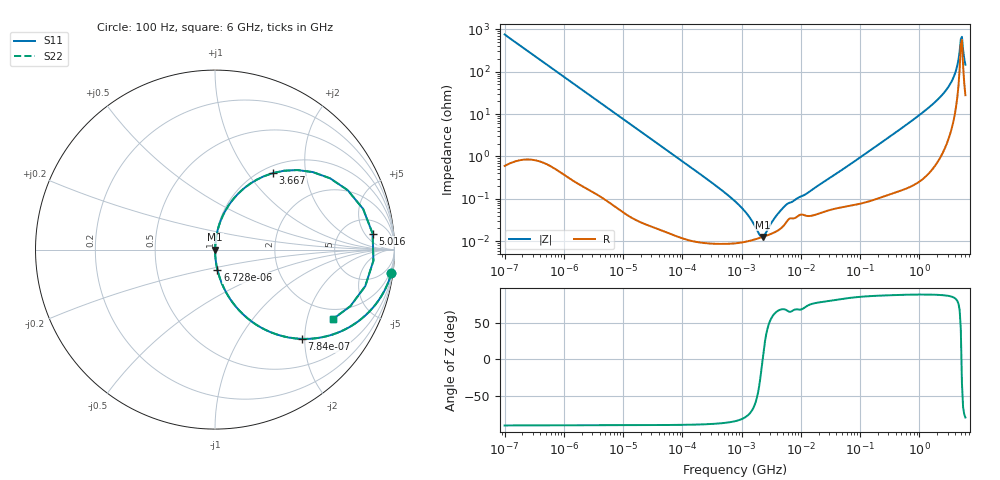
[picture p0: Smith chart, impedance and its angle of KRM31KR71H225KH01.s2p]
!Murata Part Number: KRM31KR71H225KH01
!These Parameters are Measured in Series Mode Connection
!Data Generated on Jan 08, 2026
!  o--ll--o
!Port1  Port2
!  o------o
!Operation Temp=25[degC], DC Bias Voltage=0[V]
!Freq. Start=100[Hz] Stop=6[GHz] 401[Steps]
# Hz S RI R 50
!Freq.(Hz) S11(Real) S11(Imag) S21(Real) S21(Imag) S12(Real) S12(Imag) S22(Real) S22(Imag)
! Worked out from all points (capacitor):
!   401 points, 100 Hz to 6 GHz, reference 50 ohm
!   read as one part in series: C = 2.11 uF near 109 Hz
!   lowest |Z| = 12.6 mohm at 2.269 MHz (marker M1)
!   series resonance near 2.264 MHz, so ESL is about 2.3 nH
!   S11 on the Smith chart (normalised r, x): 100 Hz: 1, -15; 784 Hz: 1.01, -1.93; 6.728 kHz: 1.00, -0.23; 3.667 GHz: 1.11, +1.33; 5.016 GHz: 10, +8; 6 GHz: 1.56, -2.88
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100  0.9827 -0.13  0.0173 0.13  0.0173 0.13  0.9827 -0.13
293  0.8688 -0.336  0.1312 0.336  0.1312 0.336  0.8688 -0.336
784  0.4836 -0.4973  0.5164 0.4973  0.5164 0.4973  0.4836 -0.4973
2008  0.1269 -0.3302  0.8731 0.3302  0.8731 0.3302  0.1269 -0.3302
6728  0.0134 -0.1121  0.9866 0.1121  0.9866 0.1121  0.0134 -0.1121
40335  0.000553 -0.019  0.9994 0.019  0.9994 0.019  0.000553 -0.019
774597  9e-05 -0.000875  0.9999 0.000875  0.9999 0.000875  9e-05 -0.000875
1212075  9.85e-05 -0.000446  0.9999 0.000446  0.9999 0.000446  9.85e-05 -0.000446
1983483  0.000119 -8.69e-05  0.9999 8.69e-05  0.9999 8.69e-05  0.000119 -8.69e-05
2268635  0.000126 1.5e-06  0.9999 -1.5e-06  0.9999 -1.5e-06  0.000126 1.5e-06
5311619  0.000247 0.000619  0.9998 -0.000619  0.9998 -0.000619  0.000247 0.000619
1.555665e7  0.000404 0.00159  0.9996 -0.00159  0.9996 -0.00159  0.000404 0.00159
3.124326e8  0.00209 0.0288  0.9979 -0.0288  0.9979 -0.0288  0.00209 0.0288
9.569533e8  0.0104 0.089  0.9896 -0.089  0.9896 -0.089  0.0104 0.089
2.048624e9  0.0528 0.2072  0.9472 -0.2072  0.9472 -0.2072  0.0528 0.2072
2.931063e9  0.1454 0.3272  0.8546 -0.3272  0.8546 -0.3272  0.1454 0.3272
3.666503e9  0.3223 0.4263  0.6777 -0.4263  0.6777 -0.4263  0.3223 0.4263
4.385646e9  0.6412 0.3973  0.3588 -0.3973  0.3588 -0.3973  0.6412 0.3973
4.796499e9  0.8253 0.2263  0.1747 -0.2263  0.1747 -0.2263  0.8253 0.2263
5.016141e9  0.8781 0.0895  0.1219 -0.0895  0.1219 -0.0895  0.8781 0.0895
5.486059e9  0.837 -0.2038  0.163 0.2038  0.163 0.2038  0.837 -0.2038
6e9  0.6554 -0.3883  0.3446 0.3883  0.3446 0.3883  0.6554 -0.3883
